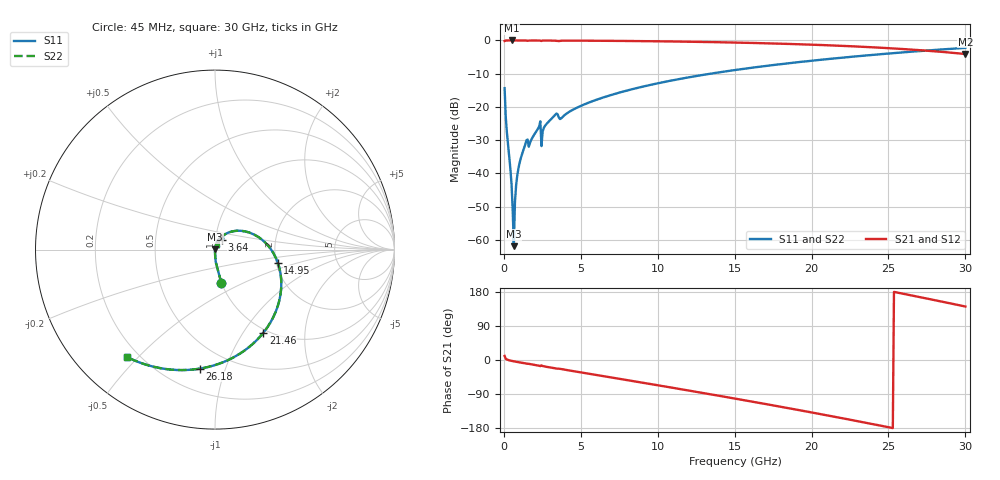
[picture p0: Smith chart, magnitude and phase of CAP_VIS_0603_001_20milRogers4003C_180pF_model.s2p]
! S-parameter model data by Modelithics Inc.  support@modelithics.com  813-866-6335  Tampa FL USA
! S-Parameter data specifications:
! Substrate: 20-mil Rogers 4003C, substrate thickness, H=0.508mm, Dielectric constant, Er=3.75
! PCB Mounting Pad Footprint: Pad width, PadW=0.90mm , Pad length, PadL=1.00mm , Pad gap, PadG (edge-to-edge)=1.00mm , Reference planes=3.0mm apart
! Created Wed Nov 18 13:32:42 2015
# hz S ma R 50
! 2 Port Network Data from SP1.SP block
! freq  magS11  angS11  magS21  angS21  magS12  angS12  magS22  angS22
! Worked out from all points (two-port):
!   401 points, 45 MHz to 30 GHz, reference 50 ohm
!   highest |S21| = 0.00 dB at 494.3 MHz (marker M1); lowest = -4.1 dB at 30 GHz (marker M2)
!   |S21| within 3 dB of the highest: start of sweep to 27.26 GHz
!   lowest |S11| = -61.9 dB at 644.1 MHz (marker M3), VSWR 1.00, Z = 50.1 + j0.0584 ohm
!   |S11| at or under -10 dB: start of sweep to 13.44 GHz
!   |S22| runs from -61.9 to -2.2 dB; largest |S21 - S12| = 0
!   S11 on the Smith chart (normalised r, x): 45 MHz: 1.00, -0.39; 3.64 GHz: 1.07, +0.12; 14.95 GHz: 2.04, -0.34; 21.46 GHz: 0.95, -1.24; 26.18 GHz: 0.34, -0.82; 30 GHz: 0.16, -0.47
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4.5e7  0.1915 -79.1  0.9813 10.8  0.9813 10.8  0.1915 -79.1
3.4455e8  0.01799 -89.6  0.9994 -0.8  0.9994 -0.8  0.01799 -89.6
4.94325e8  0.006913 -88.5  0.9995 -2.3  0.9995 -2.3  0.006913 -88.5
6.441e8  0.0008026 46.6  0.9994 -3.5  0.9994 -3.5  0.0008026 46.6
7.93875e8  0.006632 80.4  0.9993 -4.6  0.9993 -4.6  0.006632 80.4
8.687625e8  0.009314 81.1  0.9993 -5.2  0.9993 -5.2  0.009314 81.1
1.018538e9  0.01434 81.1  0.9991 -6.3  0.9991 -6.3  0.01434 81.1
1.392975e9  0.02741 77.8  0.998 -9.0  0.998 -9.0  0.02741 77.8
1.767412e9  0.03162 75.8  0.9978 -11.3  0.9978 -11.3  0.03162 75.8
2.216738e9  0.047 73.8  0.9974 -14.6  0.9974 -14.6  0.047 73.8
2.591175e9  0.04821 71.6  0.9971 -16.7  0.9971 -16.7  0.04821 71.6
3.265162e9  0.07301 64.9  0.9927 -21.7  0.9927 -21.7  0.07301 64.9
3.6396e9  0.06561 55.2  0.9844 -23.2  0.9844 -23.2  0.06561 55.2
5.062462e9  0.1051 55.9  0.9923 -33.1  0.9923 -33.1  0.1051 55.9
1.007992e10  0.2285 22.3  0.9707 -67.2  0.9707 -67.2  0.2285 22.3
1.494761e10  0.3568 -11.7  0.9304 -101.3  0.9304 -101.3  0.3568 -11.7
1.50225e10  0.3588 -12.2  0.9296 -101.8  0.9296 -101.8  0.3588 -12.2
2.003996e10  0.4962 -49.0  0.8632 -138.7  0.8632 -138.7  0.4962 -49.0
2.146282e10  0.5358 -59.8  0.8389 -149.5  0.8389 -149.5  0.5358 -59.8
2.505742e10  0.637 -88.2  0.7643 -177.9  0.7643 -177.9  0.637 -88.2
2.618074e10  0.6686 -97.3  0.7365 173.0  0.7365 173.0  0.6686 -97.3
3e10  0.7731 -129.1  0.6252 141.2  0.6252 141.2  0.7731 -129.1
